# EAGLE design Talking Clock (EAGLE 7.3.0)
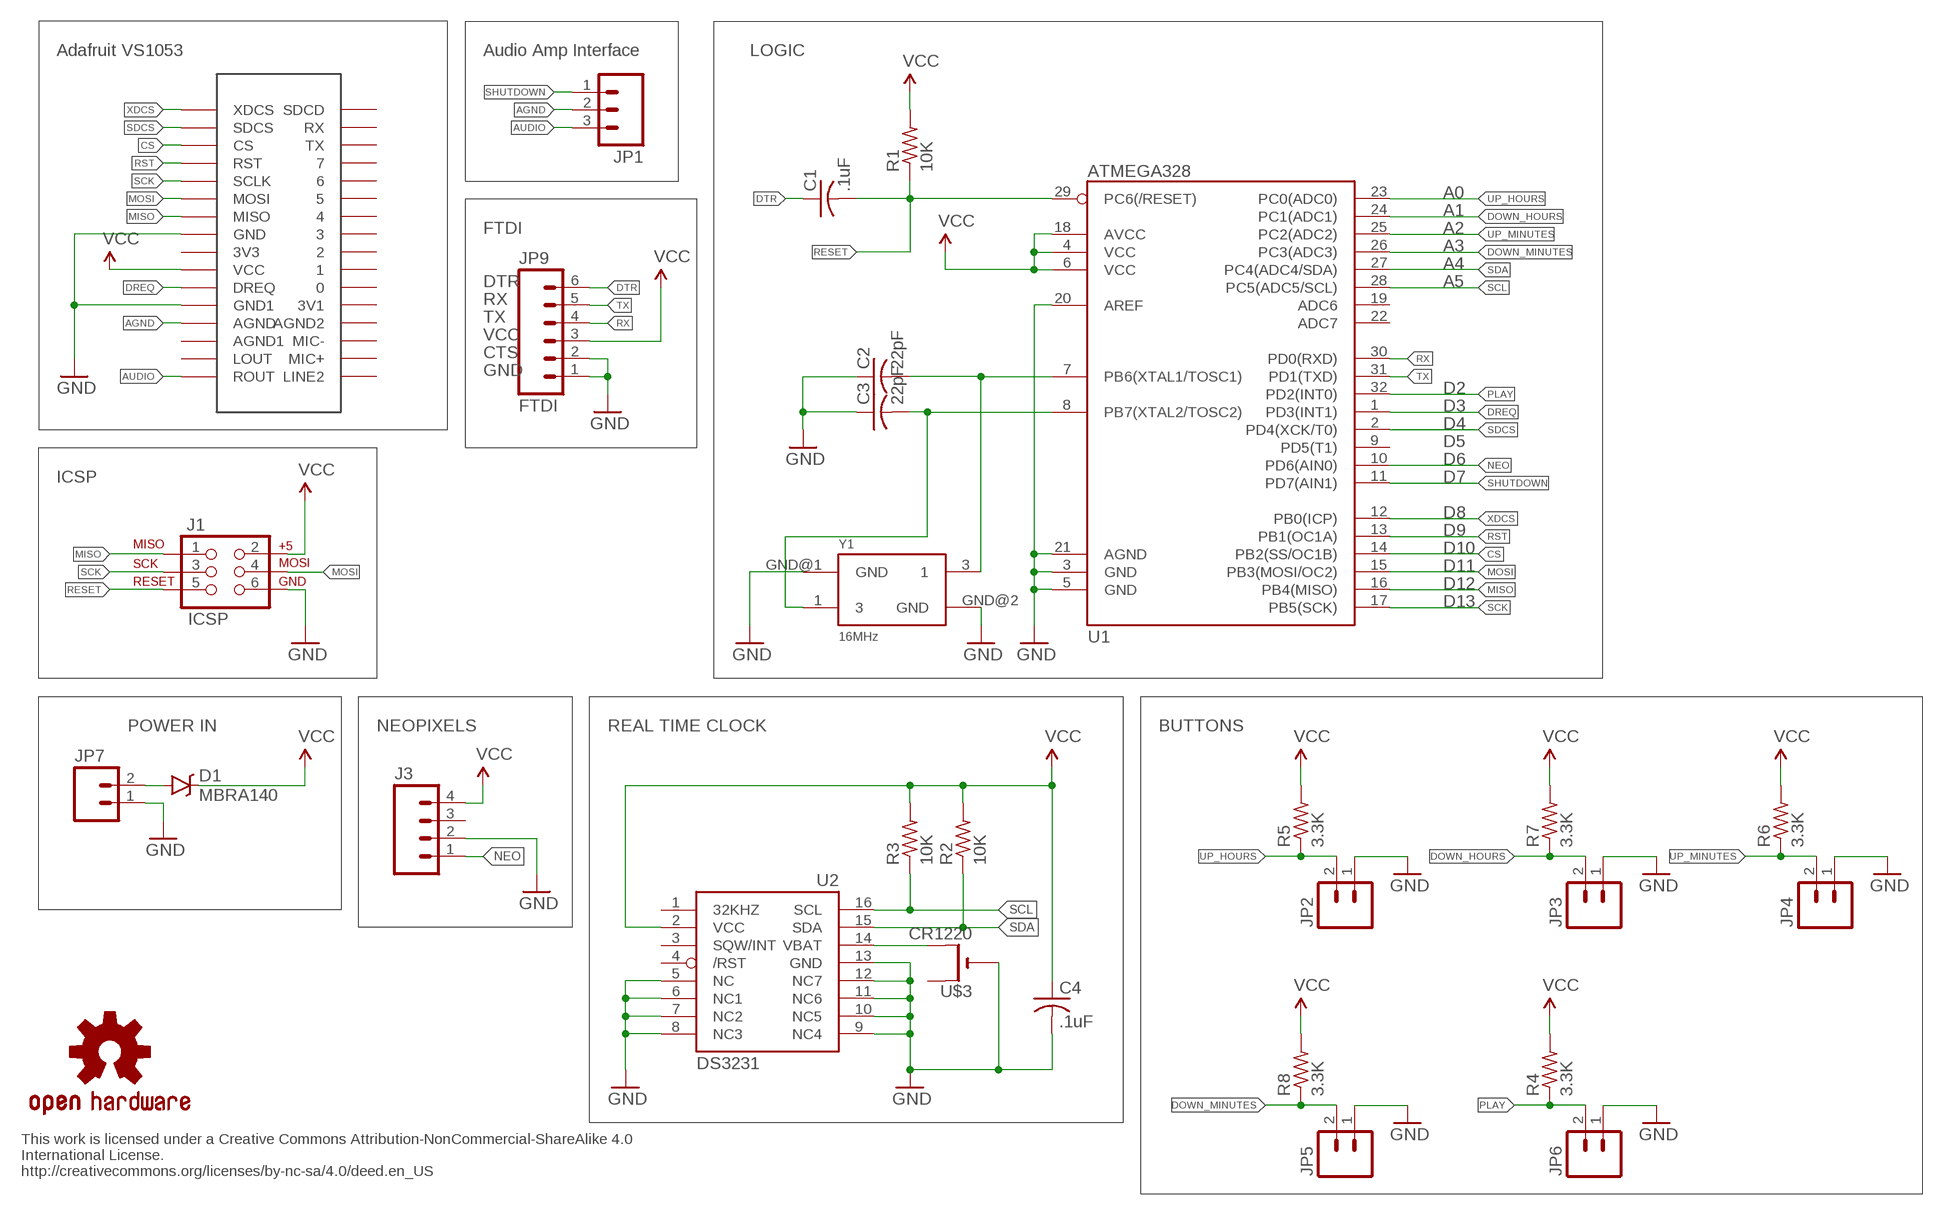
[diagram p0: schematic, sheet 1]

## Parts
C1  .1uF  C-USC0805K  [C0805K]
C2  22pF  C-USC0805K  [C0805K]
C3  22pF  C-USC0805K  [C0805K]
C4  .1uF  C-USC0805K  [C0805K]
D1  MBRA140  [SMA-DIODE]
J1  ICSP  AVR_SPI_PRG_6PTH  [2X3]
J3  M04PTH  [1X04]
JP1  M03PTH  [1X03]
JP2  M02PTH  [1X02]
JP3  M02PTH  [1X02]
JP4  M02PTH  [1X02]
JP5  M02PTH  [1X02]
JP6  M02PTH  [1X02]
JP7  M02PTH  [1X02]
JP9  FTDI  M06NO_SILK_FEMALE_PTH  [1X06_NO_SILK]
R1  10K  R-US_R0805  [R0805]
R2  10K  R-US_R0805  [R0805]
R3  10K  R-US_R0805  [R0805]
R4  3.3K  R-US_R0805  [R0805]
R5  3.3K  R-US_R0805  [R0805]
R6  3.3K  R-US_R0805  [R0805]
R7  3.3K  R-US_R0805  [R0805]
R8  3.3K  R-US_R0805  [R0805]
U1  ATMEGA328  ATMEGA328_SMT  [TQFP32-08]
U2  DS3231  DS3231/SO  [SO16W]
U$1  ADAFRUIT_V1503  [ADAFRUITVS1053]
U$3  CR1220  CR1220SMT  [CR1220-SMD]
U$7  OSHW-LOGOS  [OSHW-LOGO-S]
Y1  16MHz  OSCILLATOR5X3  [CRYSTAL-SMD-5X3]

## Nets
AGND: JP1.2 U$1.P$13(AGND)
AUDIO: JP1.3 U$1.P$16(ROUT)
CS: U1.14(PB2(SS/OC1B)) U$1.P$3(CS)
DOWN_HOURS: JP3.2 R7.1 U1.24(PC1(ADC1))
DOWN_MINUTES: JP5.2 R8.1 U1.26(PC3(ADC3))
DREQ: U1.1(PD3(INT1)) U$1.P$11(DREQ)
DTR: C1.1 JP9.6
GND: C2.1 C3.1 C4.2 J1.6 J3.2 JP2.1 JP3.1 JP4.1 JP5.1 JP6.1 JP7.1 JP9.1 JP9.2 U1.3(GND) U1.5(GND) U1.20(AREF) U1.21(AGND) U2.5(NC) U2.6(NC1) U2.7(NC2) U2.8(NC3) U2.9(NC4) U2.10(NC5) U2.11(NC6) U2.12(NC7) U2.13(GND) U$1.P$8(GND) U$1.P$12(GND1) U$3.- Y1.GND@1(GND) Y1.GND@2(GND)
MISO: J1.1 U1.16(PB4(MISO)) U$1.P$7(MISO)
MOSI: J1.4 U1.15(PB3(MOSI/OC2)) U$1.P$6(MOSI)
N$4: D1.A JP7.2
N$8: C3.2 U1.8(PB7(XTAL2/TOSC2)) Y1.1
N$10: C2.2 U1.7(PB6(XTAL1/TOSC1)) Y1.3
N$141: U2.14(VBAT) U$3.+$2(+1)
NEO: J3.1 U1.10(PD6(AIN0))
PLAY: JP6.2 R4.1 U1.32(PD2(INT0))
RESET: C1.2 J1.5 R1.1 U1.29(PC6(/RESET))
RST: U1.13(PB1(OC1A)) U$1.P$4(RST)
RX: JP9.4 U1.30(PD0(RXD))
SCK: J1.3 U1.17(PB5(SCK)) U$1.P$5(SCLK)
SCL: R3.1 U1.28(PC5(ADC5/SCL)) U2.16(SCL)
SDA: R2.1 U1.27(PC4(ADC4/SDA)) U2.15(SDA)
SDCS: U1.2(PD4(XCK/T0)) U$1.P$2(SDCS)
SHUTDOWN: JP1.1 U1.11(PD7(AIN1))
TX: JP9.5 U1.31(PD1(TXD))
UP_HOURS: JP2.2 R5.1 U1.23(PC0(ADC0))
UP_MINUTES: JP4.2 R6.1 U1.25(PC2(ADC2))
VCC: C4.1 D1.C J1.2 J3.4 JP9.3 R1.2 R2.2 R3.2 R4.2 R5.2 R6.2 R7.2 R8.2 U1.4(VCC) U1.6(VCC) U1.18(AVCC) U2.2(VCC) U$1.P$10(VCC)
XDCS: U1.12(PB0(ICP)) U$1.P$1(XDCS)
Unconnected: J3.3 U1.9(PD5(T1)) U1.19(ADC6) U1.22(ADC7) U2.1(32KHZ) U2.3(SQW/INT) U2.4(/RST) U$1.P$9(3V3) U$1.P$14(AGND1) U$1.P$15(LOUT) U$1.P$17(LINE2) U$1.P$18(MIC+) U$1.P$19(MIC-) U$1.P$20(AGND2) U$1.P$21(3V1) U$1.P$22 U$1.P$23 U$1.P$24 U$1.P$25 U$1.P$26 U$1.P$27 U$1.P$28 U$1.P$29 U$1.P$30(TX) U$1.P$31(RX) U$1.P$32(SDCD) U$3.+$1(+)

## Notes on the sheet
- Adafruit VS1053 | Audio Amp Interface | LOGIC
- A0
- A1
- FTDI | A2
- A3
- A4
- DTR | A5
- RX
- TX
- VCC
- CTS
- GND
- D2
- D3
- D4
- D5
- D6
- ICSP | D7
- D8
- D9
- D10
- D11
- D12
- D13
- POWER IN | NEOPIXELS | REAL TIME CLOCK | BUTTONS
- This work is licensed under a Creative Commons Attribution-NonCommercial-ShareAlike 4.0
  International License.
  http://creativecommons.org/licenses/by-nc-sa/4.0/deed.en_US

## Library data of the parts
C1-C4 = adafruit:C-US: CAPACITOR, American symbol
D1 = SparkFun-DiscreteSemi:MBRA140: 40V, 1A Schottky rectifier; PROD_ID: DIO-08053
J1 = SparkFun:AVR_SPI_PRG_6: AVR ISP 6 Pin This is the reduced ISP connector for AVR programming. Common on Arduino. This footprint will take up less PCB space and can be used with a 10-pin to 6-pin adapter such as SKU: BOB-08508; OC_NEWARK: unknown
J3 = SparkFun-Connectors:M04: Header 4 Standard 4-pin 0.1" header. Use with straight break away headers (SKU : PRT-00116), right angle break away headers (PRT-00553), swiss pins (PRT-00743), machine pins (PRT-00117), and female headers (PRT-00115). Molex polarized connector foot print use with SKU : PRT-08231 with associated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; PROD_ID: CONN-09696
JP1 = SparkFun-Connectors:M03: Header 3 Standard 3-pin 0.1" header. Use with straight break away headers (SKU : PRT-00116), right angle break away headers (PRT-00553), swiss pins (PRT-00743), machine pins (PRT-00117), and female headers (PRT-00115). Molex polarized connector foot print use with SKU : PRT-08232 with associated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
JP2-JP7 = SparkFun-Connectors:M02: Standard 2-pin 0.1" header. Use with
JP9 = SparkFun-Connectors:M06: Header 6 Standard 6-pin 0.1" header. Use with straight break away headers (SKU : PRT-00116), right angle break away headers (PRT-00553), swiss pins (PRT-00743), machine pins (PRT-00117), and female headers (PRT-00115). Molex polarized connector foot print use with SKU : PRT-08094 with associated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; PROD_ID: CONN-08437
R1-R8 = adafruit:R-US_: RESISTOR, American symbol
U1 = SparkFun-DigitalIC:ATMEGA328_SMT: 32-Pin Atmega328 part Commonly used on Arduino compatible boards Available in QFP and QFN packages TQFP is IC-09069 QFN is non-stock; PROD_ID: IC-09069; VALUE: ATMEGA328P
U2 = adafruit:DS3231
U$1 = Adafruit VS1053:ADAFRUIT_V1503
U$3 = adafruit:CR1220: CR1216/CR1220/CR1225 12mm 3V lithium coin cell Great for battery packup. Both SMT and THM holders. Note the THM package has the ground pads on both sides of the PCB so that the masks are the same - this reduces the cost
U$7 = SparkFun:OSHW-LOGO: Open Source Hardware Logo This logo indicates the piece of hardware it is found on incorporates a OSHW license and/or adheres to the definition of open source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
Y1 = SparkFun-FreqCtrl:OSCILLATOR: Generic 5x3 and 7x5 oscillators

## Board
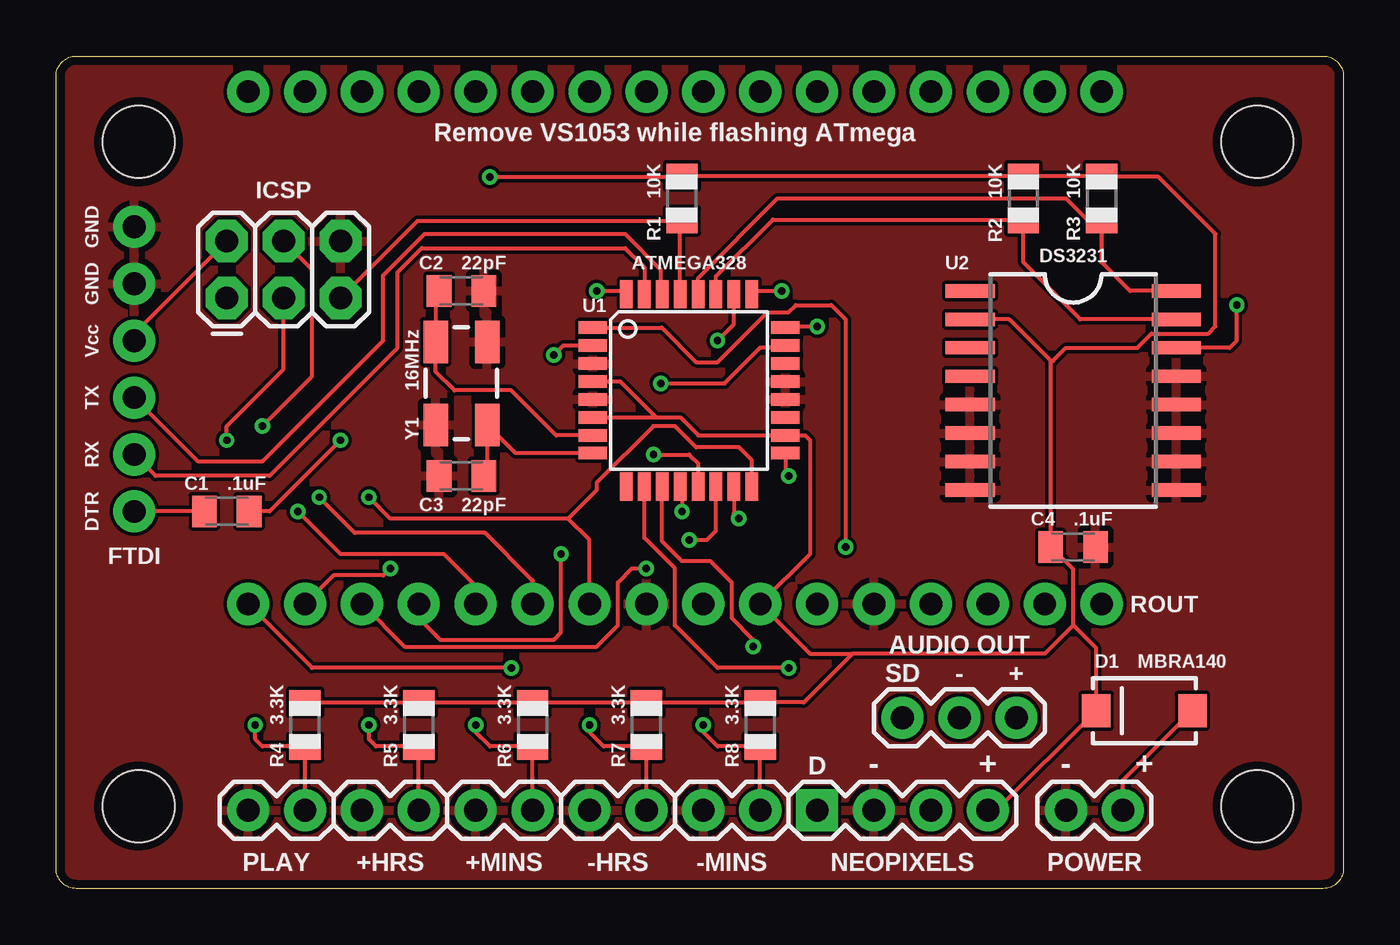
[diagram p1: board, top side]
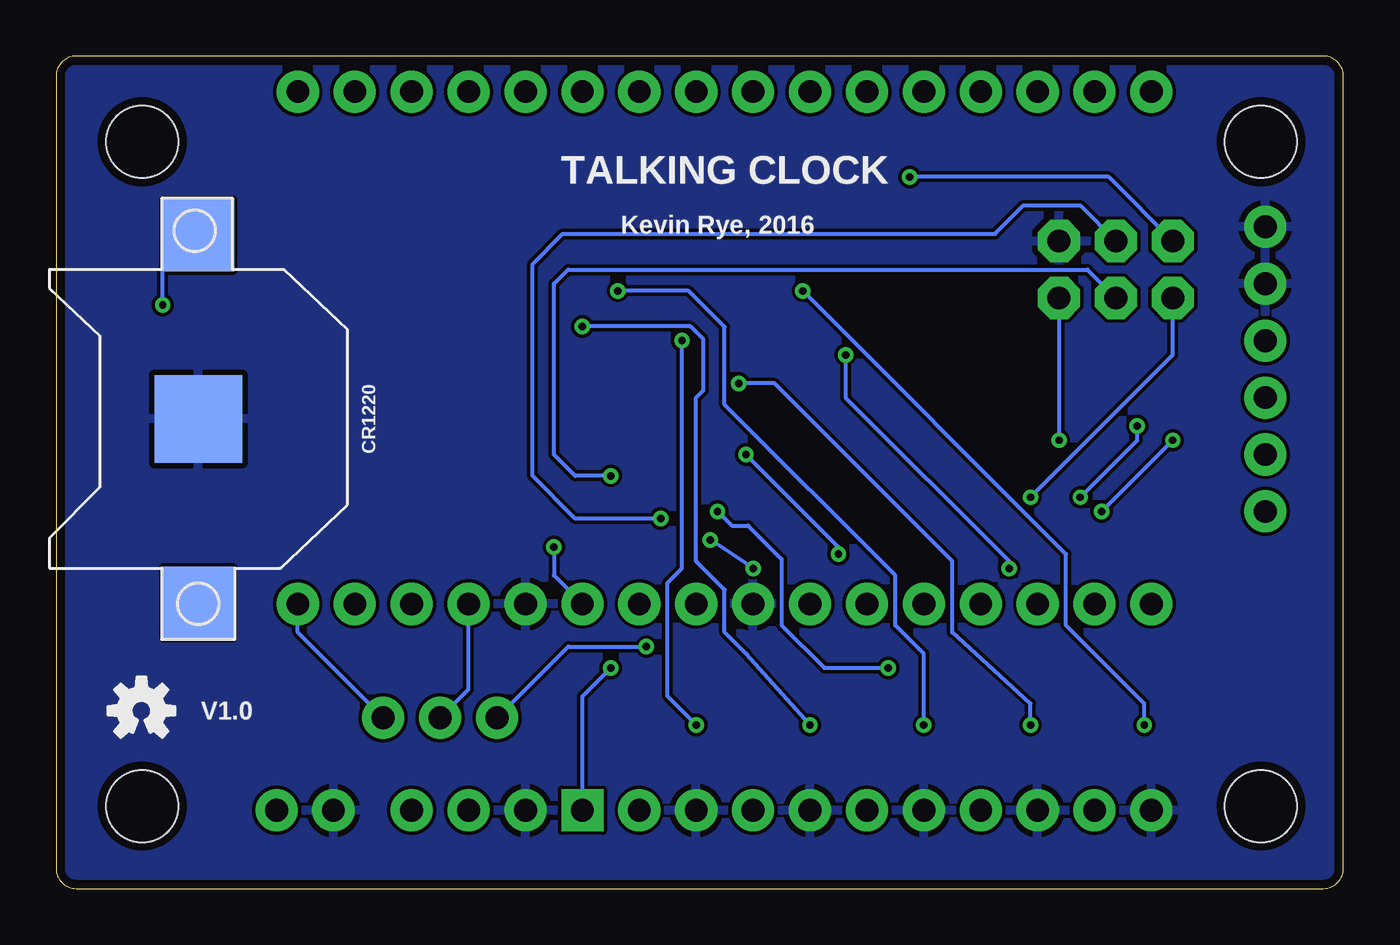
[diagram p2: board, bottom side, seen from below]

Size 57.47 x 37.15 mm. Coordinates in mm from the lower left corner, seen from the top.
Outline: 0.9,37.15 56.57,37.15 arc-90 57.47,36.25 57.47,0.9 arc-90 56.57,0 0.9,0 arc-90 0,0.9 0,36.25 arc-90 0.9,37.15
Copper layers (1*16): Top 0.0356mm / dielectric 1.5011mm / Bottom 0.0356mm
Design rules "LaenPCBOrder": minimum track width 6mil, minimum drill 13mil, track to track 6mil, track to pad 6mil, pad to pad 6mil, via to via 6mil, smd to smd 6mil, copper to edge 15mil, drill to drill 6mil, minimum pad ring 7mil, minimum via ring 7mil, stop-mask expansion 3mil, vias tented up to drill 0mil, thermal gap 10mil
Holes 3.2 mm at 3.68,33.32 3.68,3.68 53.62,3.68 53.62,33.32

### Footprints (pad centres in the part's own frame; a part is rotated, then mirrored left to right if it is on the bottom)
C0805K = smd 1.1 x 1.4: 1 -1,0; 2 1,0
SMA-DIODE = smd 1.27 x 1.47: A -2.15,0; C 2.15,0
2X3 = drill 1.016 pad 1.88 octagon: 1 0,0; 2 0,2.54; 3 2.54,0; 4 2.54,2.54; 5 5.08,0; 6 5.08,2.54
1X04 = drill 1.016 pad 1.88 square: 1 0,0 | drill 1.016 pad 1.88: 2 2.54,0; 3 5.08,0; 4 7.62,0
1X03 = drill 1.016 pad 1.88: 1 0,0; 2 2.54,0; 3 5.08,0
1X02 = drill 1.016 pad 1.88: 1 0,0; 2 2.54,0
1X06_NO_SILK = drill 1.016 pad 1.88: 1 0,0; 2 2.54,0; 3 5.08,0; 4 7.62,0; 5 10.16,0; 6 12.7,0
R0805 = smd 1.1 x 1.4: 1 -1,0; 2 1,0
TQFP32-08 = smd 1.27 x 0.559: 1 -4.293,2.8; 2 -4.293,2; 3 -4.293,1.2; 4 -4.293,0.4; 5 -4.293,-0.4; 6 -4.293,-1.2; 7 -4.293,-2; 8 -4.293,-2.8; 17 4.293,-2.8; 18 4.293,-2; 19 4.293,-1.2; 20 4.293,-0.4; 21 4.293,0.4; 22 4.293,1.2; 23 4.293,2; 24 4.293,2.8 | smd 0.559 x 1.27: 9 -2.8,-4.293; 10 -2,-4.293; 11 -1.2,-4.293; 12 -0.4,-4.293; 13 0.4,-4.293; 14 1.2,-4.293; 15 2,-4.293; 16 2.8,-4.293; 25 2.8,4.293; 26 2,4.293; 27 1.2,4.293; 28 0.4,4.293; 29 -0.4,4.293; 30 -1.2,4.293; 31 -2,4.293; 32 -2.8,4.293
SO16W = smd 0.6 x 2.2: 1 -4.445,-4.6; 2 -3.175,-4.6; 3 -1.905,-4.6; 4 -0.635,-4.6; 5 0.635,-4.6; 6 1.905,-4.6; 7 3.175,-4.6; 8 4.445,-4.6; 9 4.445,4.6; 10 3.175,4.6; 11 1.905,4.6; 12 0.635,4.6; 13 -0.635,4.6; 14 -1.905,4.6; 15 -3.175,4.6; 16 -4.445,4.6
ADAFRUITVS1053 = drill 1.016 pad 1.88: P$1 8.89,2.54; P$2 11.43,2.54; P$3 13.97,2.54; P$4 16.51,2.54; P$5 19.05,2.54; P$6 21.59,2.54; P$7 24.13,2.54; P$8 26.67,2.54; P$9 29.21,2.54; P$10 31.75,2.54; P$11 34.29,2.54; P$12 36.83,2.54; P$13 39.37,2.54; P$14 41.91,2.54; P$15 44.45,2.54; P$16 46.99,2.54; P$17 46.99,25.4; P$18 44.45,25.4; P$19 41.91,25.4; P$20 39.37,25.4; P$21 36.83,25.4; P$22 34.29,25.4; P$23 31.75,25.4; P$24 29.21,25.4; P$25 26.67,25.4; P$26 24.13,25.4; P$27 21.59,25.4; P$28 19.05,25.4; P$29 16.51,25.4; P$30 13.97,25.4; P$31 11.43,25.4; P$32 8.89,25.4
CR1220-SMD = smd 3.2 x 3.2: +$1 -8.2,0; +$2 8.2,0 | smd 3.9 x 3.9: - 0,0
CRYSTAL-SMD-5X3 = smd 1.9 x 1.1: 1 -1.85,-1.15; 3 1.85,1.15; GND@1 -1.85,1.15; GND@2 1.85,-1.15

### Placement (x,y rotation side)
C1  7.62,16.83 0 top
C2  18.1,26.67 180 top
C3  18.1,18.41 0 top
C4  45.4,15.24 0 top
D1  48.58,7.94 180 top
J1  7.62,26.35 0 top
J3  33.97,3.49 0 top
JP1  37.78,7.62 0 top
JP2  13.65,3.49 0 top
JP3  23.81,3.49 0 top
JP4  18.73,3.49 0 top
JP5  28.89,3.49 0 top
JP6  8.57,3.49 0 top
JP7  45.09,3.49 0 top
JP9  3.49,29.53 270 top
R1  27.94,30.8 90 top
R2  43.18,30.8 90 top
R3  46.67,30.8 90 top
R4  11.11,7.3 90 top
R5  16.19,7.3 90 top
R6  21.27,7.3 90 top
R7  26.35,7.3 90 top
R8  31.43,7.3 90 top
U1  28.26,22.23 0 top
U2  45.4,22.23 270 top
U$1  -0.32,10.16 0 top
U$3  51.12,20.95 90 bottom
U$7  53.66,7.94 0 bottom
Y1  18.1,22.54 90 top

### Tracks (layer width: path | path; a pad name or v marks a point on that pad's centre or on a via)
AGND
  Bottom 0.178: JP1.2 39.05,8.89 U$1.P$13
AUDIO
  Bottom 0.178: JP1.3 46.67,11.43 U$1.P$16
CS  (via drill 0.33)
  Top 0.178: U$1.P$3 15.56,10.79 24.13,10.79 25.08,11.75 25.08,13.65 25.72,14.29 v26.35,14.29 | v28.26,15.56 29.05,15.56 29.46,15.96 U1.14
  Bottom 0.178: v26.35,14.29 v28.26,15.56
DOWN_HOURS  (via drill 0.33)
  Top 0.178: JP3.2 R7.1 26.3,6.35 24.45,6.35 23.81,6.99 v23.81,7.3 | U1.24 32.61,25.08 v33.97,25.08
  Bottom 0.178: v23.81,7.3 26.67,10.48 27.62,11.43 27.62,13.34 28.89,14.61 28.89,21.91 28.57,22.23 28.57,24.5 29.16,25.08 v33.97,25.08
DOWN_MINUTES  (via drill 0.33)
  Top 0.178: JP5.2 R8.1 31.39,6.35 29.53,6.35 28.89,6.99 v28.89,7.3 | U1.26 30.26,25.18 v29.53,24.45
  Bottom 0.178: v29.53,24.45 29.53,14.29 30.16,13.65 30.16,8.57 v28.89,7.3
DREQ  (via drill 0.33)
  Top 0.178: U1.1 27.05,25.02 28.57,23.5 29.53,23.5 31.75,25.72 32.7,25.72 33.02,26.04 34.61,26.04 35.24,25.4 v35.24,15.24
  Bottom 0.178: v35.24,15.24 35.24,13.97 U$1.P$11
DTR
  Top 0.178: C1.1 JP9.6
GND
  pour Top: -1.27,38.42 58.42,38.73 58.42,-0.64 -1.27,-0.64
  pour Bottom: -2.22,39.37 59.37,39.37 59.37,-1.27 -2.22,-1.59
MISO  (via drill 0.33)
  Top 0.178: U$1.P$7 23.81,15.56 22.86,16.51 | 22.86,16.51 14.92,16.51 v13.97,17.46 | U1.16 31.06,19.11 30.48,19.68 28.57,19.68 27.62,20.64 26.67,20.64 24.13,18.1 24.13,17.78 22.86,16.51
  Bottom 0.178: v13.97,17.46 7.62,23.81 J1.1
MOSI  (via drill 0.33)
  Top 0.178: U$1.P$6 21.27,13.74 19.14,15.88 13.34,15.88 v11.75,17.46 | v9.21,20.64 11.43,22.86 11.43,27.62 J1.4 | U1.15 30.26,16.73 v30.48,16.51
  Bottom 0.178: v11.75,17.46 9.21,20 v9.21,20.64 | v30.48,16.51 34.29,16.51 36.2,18.41 36.2,27.86 34.85,29.21 15.56,29.21 14.29,30.48 11.75,30.48 J1.4
N$4
  Top 0.178: JP7.2 47.62,4.83 D1.A
N$8
  Top 0.178: U1.8 20.52,19.43 Y1.1 19.25,18.41 C3.2 19.41,18.41
N$10
  Top 0.178: 17.1,24.54 Y1.3 | U1.7 22.32,20.23 20.32,22.23 17.78,22.23 16.95,23.06 Y1.3 | C2.2 16.95,26.67 Y1.3
N$141  (via drill 0.33)
  Top 0.178: U2.14 52.39,24.13 52.7,24.45 v52.7,26.04
  Bottom 0.178: 51.12,27.62 U$3.+$2 52.7,27.57 v52.7,26.04
NEO  (via drill 0.33)
  Top 0.178: v32.7,9.84 29.53,9.84 27.62,11.75 27.62,14.29 26.26,15.65 U1.10
  Bottom 0.178: J3.1 33.97,8.57 v32.7,9.84
PLAY  (via drill 0.33)
  Top 0.178: JP6.2 R4.1 11.06,6.35 9.21,6.35 8.89,6.67 v8.89,7.3 | 25.4,26.46 U1.32 25.3,26.67 v24.13,26.67
  Bottom 0.178: v8.89,7.3 8.89,8.26 12.38,11.75 12.38,14.92 v24.13,26.67
RESET  (via drill 0.33)
  Top 0.178: U1.29 27.86,29.71 R1.1 16.14,29.8 J1.5 | v12.7,20 9.53,16.83 C1.2
  Bottom 0.178: J1.5 v12.7,20
RST  (via drill 0.33)
  Top 0.178: U$1.P$4 16.19,12.06 17.14,11.11 22.23,11.11 22.54,11.43 v22.54,14.92 | v26.67,19.37 28.26,19.37 28.66,18.97 U1.13
  Bottom 0.178: v22.54,14.92 22.54,15.24 v26.67,19.37
RX
  Top 0.178: U1.30 26.99,26.59 26.99,27.62 25.4,29.21 16.46,29.21 14.61,27.36 14.61,24.45 9.21,19.05 6.35,19.05 JP9.4
SCK  (via drill 0.33)
  Top 0.178: U$1.P$5 18.73,13.5 17.31,14.92 12.7,14.92 v10.79,16.83 | v7.62,20 7.62,20.64 10.16,23.18 J1.3 | U1.17 32.55,18.57 v32.7,18.41
  Bottom 0.178: v10.79,16.83 v7.62,20 | v32.7,18.41 34.29,18.41 35.24,19.37 35.24,26.99 34.61,27.62 11.43,27.62 J1.3
SCL
  Top 0.178: U2.16 47.94,26.67 46.67,27.94 R3.1 46.09,29.8 45.09,30.8 32.21,30.8 28.66,27.24 U1.28
SDA
  Top 0.178: U2.15 45.72,25.4 43.18,27.94 R2.1 43.13,29.84 31.99,29.84 29.46,27.31 U1.27
SDCS  (via drill 0.33)
  Top 0.178: U1.2 22.64,24.23 v22.23,23.81 | v14.92,14.29 14.61,13.97 12.38,13.97 U$1.P$2
  Bottom 0.178: v22.23,23.81 22.23,21.91 14.92,14.61 v14.92,14.29
SHUTDOWN  (via drill 0.33)
  Top 0.178: 26.99,17.93 U1.11 27.06,15.49 27.94,14.61 29.21,14.61 30.16,13.65 30.16,12.06 31.11,11.11 v31.11,10.79
  Bottom 0.178: JP1.1 34.61,10.79 v31.11,10.79
TX
  Top 0.178: U1.31 26.26,27.72 25.4,28.57 16.32,28.57 15.24,27.49 15.24,24.13 9.53,18.41 4.45,18.41 JP9.5
UP_HOURS  (via drill 0.33)
  Top 0.178: JP2.2 R5.1 16.14,6.35 14.29,6.35 13.97,6.67 v13.97,7.3 | v26.99,22.54 29.84,22.54 31.43,24.13 32.45,24.13 U1.23
  Bottom 0.178: v13.97,7.3 13.97,8.26 17.46,11.43 17.46,14.61 25.4,22.54 v26.99,22.54
UP_MINUTES  (via drill 0.33)
  Top 0.178: JP4.2 R6.1 21.23,6.35 19.37,6.35 18.73,6.99 v18.73,7.3 | U1.25 31.11,26.46 31.32,26.67 v32.38,26.67
  Bottom 0.178: v18.73,7.3 18.73,10.48 20,11.75 20,13.97 27.62,21.59 27.62,25.06 29.23,26.67 v32.38,26.67
VCC  (via drill 0.33)
  Top 0.178: 44.4,23.54 C4.1 45.4,14.24 45.4,11.75 | 44.4,23.54 42.55,25.4 U2.2 | 44.4,23.54 44.5,23.54 45.09,24.13 48.26,24.13 48.9,24.77 51.44,24.77 51.75,25.08 51.75,29.21 49.21,31.75 46.72,31.75 R3.2 R2.2 R1.2 27.89,31.75 v19.37,31.75 | JP9.3 3.49,24.77 J1.2 | 45.4,11.75 46.43,10.72 D1.C 41.98,3.49 J3.4 | U1.6 26.79,21.02 | 26.79,21.02 27.87,21.02 28.67,20.23 U1.18 33.43,20.23 33.66,20 33.66,14.92 U$1.P$10 33.66,10.48 35.56,10.48 | 26.79,21.02 25.19,22.62 U1.4 | 45.4,11.75 44.13,10.48 35.56,10.48 | R4.2 R5.2 R6.2 R7.2 R8.2 33.38,8.3 35.56,10.48
  Bottom 0.178: v19.37,31.75 10.48,31.75 J1.2
XDCS  (via drill 0.33)
  Top 0.178: U1.12 27.94,17.93 v27.94,16.83 | v20.32,9.84 11.43,9.84 U$1.P$1
  Bottom 0.178: v20.32,9.84 23.18,9.84 25.08,11.75 25.08,14.7 26.58,16.19 27.3,16.19 v27.94,16.83

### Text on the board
Unrouted: This work is licensed under a Creative Commons Attribution-NonCommercial-ShareAlike 4.0 International License. / http://creativecommons.org/licenses/by-nc-sa/4.0/deed.en_US
tPlace: Remove VS1053 while flashing ATmega | SD | - | + | D | - | + | - | + | +MINS | -HRS | -MINS
bPlace: TALKING CLOCK | Kevin Rye, 2016 | V1.0
tNames: GND | GND | Vcc | TX | RX | DTR | AUDIO OUT | PLAY | +HRS | NEOPIXELS | POWER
